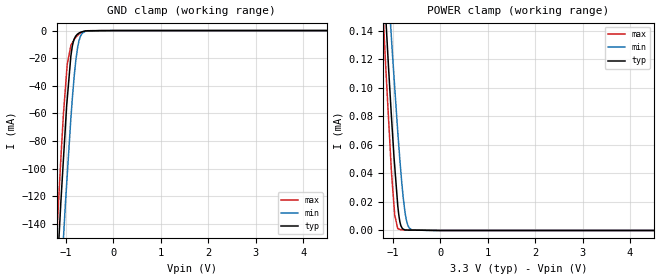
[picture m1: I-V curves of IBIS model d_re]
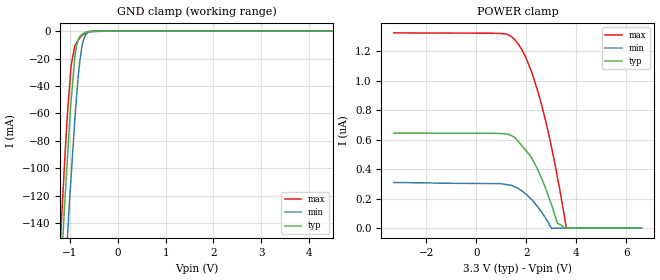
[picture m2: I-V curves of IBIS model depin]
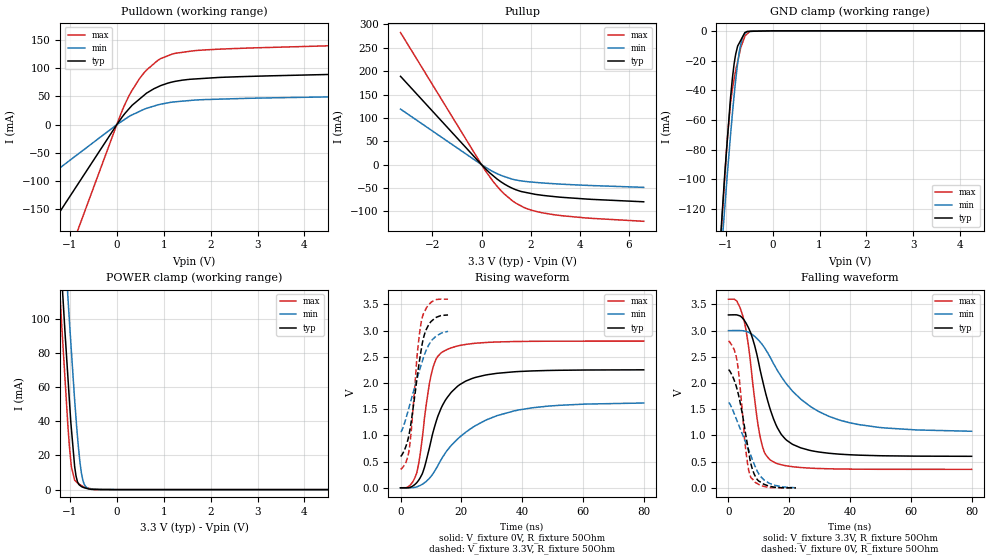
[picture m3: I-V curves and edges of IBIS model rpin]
|Texas Instruments Incorporated
| Low-Power 3.3V-supply Full-Duplex RS-485 Driver / Receiver
| Marketing part#   Digital Voltage Range   Package-type   #pins
| SN65HVD37   3V - 3.6V   D   14
[IBIS Ver]   3.2
[File name]   sn65hvd37.ibs
|SIMDE Ver   V3.0 - 201101 - RHL4 - Build 457
[File Rev]   1.0
[Date]   7/27/2011
[Source]
| Texas Instruments Incorporated.
| Analog-eLab Design Center, HPA
| 12500 TI Blvd
| Dallas, TX -75243
| e-mail: elab_scm_ibis@list.ti.com
[Notes]   Revision History:
| Rev 1.0: 7/27/2011
| - Initial version of the model
| - Model generated from simulations in TISPICE
| - Model matched to SPICE simulation
| - C_comp although listed in numerical order of value are
|   obtained from varying PVT conditions. For PVT conditions for
|   each specific value refer the buffer description under
|   respective [Model]. IBIS model user is responsible for using
|   appropriate C_comp to simulate for Signal Integrity.
|*  EXCEPTION:   *
|*  - For model d_re, there will be a leakage current in the GND   *
|*   clamp I-V Table because of the pullup on pad.   *
|*  - For model depin, there will be a leakage current in the POWER   *
|*   clamp I-V Table because of the pulldown on pad.   *
|*  - For model a_b, there will be a leakage current in both the POWER  *
|*   and GND clamp I-V Tables because of the resistor network connected*
|*   to pad.   *
|*  - For model y_z_*, there will be a leakage current in the POWER   *
|*   clamp I-V Table because of the pulldown on pad.   *
[Disclaimer]
| This model is designed as an aid for customers of Texas Instruments.
| TI and its licensors and suppliers make no warranties, either expressed
| or implied, with respect to this  model, including the warranties of
| merchantability or fitness for a particular purpose. The model is
| provided solely on an "as is" basis. The entire risk as to its quality
| and performance is with the customer.
[Copyright]
 (C) Copyright 2011 Texas Instruments Incorporated.All rights reserved.
|   SN65HVD37
[Component]   SN65HVD37
[Manufacturer]   TI
[Package]   |14 D   -  package
|   typ   min   max
R_pkg   0.05483   0.04472   0.06530
L_pkg   2.20849nH   1.82325nH   2.81275nH
C_pkg   0.42079pF   0.37741pF   0.52665pF
[Pin]  signal_name   model_name   R_pin   L_pin   C_pin
1   NC   NC   0.00380   1.93586nH  0.49616pF
2   R   rpin   0.06530   2.81275nH  0.52665pF
3   _RE   d_re   0.06113   2.26630nH  0.39911pF
4   DE   depin   0.04472   1.82325nH  0.37741pF
5   D   d_re   0.05000   1.97397nH  0.38079pF
6   GND   gnd   0.04998   2.22003nH  0.43776pF
7   GND   gnd   0.04808   2.88519nH  0.56991pF
8   NC   NC   0.00380   1.93586nH  0.49616pF
9   Y   y_z_p   0.06286   2.75675nH  0.52490pF
10   Z   y_z_n   0.05646   2.14750nH  0.39320pF
11   B   a_b   0.04527   1.84090nH  0.37881pF
12   A   a_b   0.05294   2.04647nH  0.38548pF
13   VCC   power   0.05016   2.21543nH  0.43689pF
14   VCC   power   0.04818   2.87772nH  0.56924pF
[Diff_pin]   inv_pin   vdiff   tdelay_typ   tdelay_min   tdelay_max
12   11   80mV   NA   NA   NA
9   10   NA   0   0   0
| Models and submodels in the file (6): d_re (Input), depin (Input), rpin (3-state), a_b (Input), y_z_p (3-state), y_z_n (3-state)
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|   d_re Model
[Model]   d_re
Model_type   Input
Vinl = 0.8
Vinh = 2
|   typ   min   max
|   (nom PVT)   (fast PVT)   (slow PVT)
|C_comp from frequency sweep method (F=10MHz)
|Average
|C_comp   2.050e-12   1.874e-12   2.235e-12
|C_comp from LC tank measurement(L=1nH)
|Average
|Resonant Frequency(Hz)   5.770e+09   5.890e+09   5.550e+09
C_comp   7.616e-13   7.309e-13   8.232e-13
| Where nom  PVT is Nominal Process, 3.3V, 27C
|   Fast PVT is Strong Process,  3.6V, -40C
|   Slow PVT is Weak Process,   3V, 125C
[Voltage Range]   3.3   3   3.6
|Ambient Temperature   25   85   -40
|Junction Temperature
[Temperature Range]   27   125   -40
[Power Clamp Reference]   3.3   3   3.6
[GND Clamp Reference]   0   0   0
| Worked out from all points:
|   GND clamp passes 1 mA (typ) near -0.67 V on its own axis
[GND Clamp]
|   Voltage   I(typ)   I(min)   I(max)
-3.3V     -1.705A    -1.7A      -1.738A
-1.195V   -180.4mA   -237.2mA   -148.9mA
-1.158V   -156.2mA   -213.2mA   -124.7mA
-1.112V   -126.4mA   -185.5mA   -94.94mA
-1.055V   -93.52mA   -150.9mA   -60.84mA
-975.6mV  -50.1mA    -105.4mA   -24.74mA
-897.6mV  -18.42mA   -63.54mA   -10.82mA
-858mV    -9.845mA   -45.32mA   -8.298mA
-792mV    -3.841mA   -21.25mA   -4.834mA
-693mV    -1.195mA   -3.902mA   -1.803mA
-285mV    -92.91uA   -1.638uA   -4.138uA
6.6V      0A         0A         0A
[POWER Clamp]
|   Voltage   I(typ)   I(min)   I(max)
-3.3V     1.551mA    1.444mA    1.676mA
-1.27V    222.2uA    263.9uA    196uA
-1.152V   150.7uA    198.8uA    115.5uA
-1.096V   116.7uA    169.1uA    80.94uA
-1.033V   81.39uA    136.3uA    42.71uA
-961.2mV  44.9uA     100.3uA    10.68uA
-896.4mV  17.2uA     68.68uA    1.244uA
-834.9mV  3.692uA    42.35uA    513.2nA
-744mV    365.5nA    12.7uA     396.5nA
-684mV    295nA      3.558uA    356.6nA
-591mV    254.8nA    379nA      305nA
6.6V      0A         0A         0A
|   depin Model
[Model]   depin
Model_type   Input
Vinl = 0.8
Vinh = 2.0
|   typ   min   max
|   (nom PVT)   (fast PVT)   (slow PVT)
|C_comp from frequency sweep method (F=10MHz)
|Average
|C_comp   2.070e-12   1.894e-12   2.257e-12
|C_comp from LC tank measurement(L=1nH)
|Average
|Resonant Frequency(Hz)   5.770e+09   5.890e+09   5.550e+09
C_comp   7.616e-13   7.309e-13   8.232e-13
| Where nom  PVT is Nominal Process, 3.3V, 27C
|   Fast PVT is Strong Process,  3.6V, -40C
|   Slow PVT is Weak Process,   3V, 125C
[Voltage Range]   3.3   3   3.6
|Ambient Temperature   25   85   -40
|Junction Temperature
[Temperature Range]   27   125   -40
[Power Clamp Reference]   3.3   3   3.6
[GND Clamp Reference]   0   0   0
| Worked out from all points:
|   GND clamp passes 1 mA (typ) near -0.67 V on its own axis
[GND Clamp]
|   Voltage   I(typ)   I(min)   I(max)
-3.3V     -1.705A    -1.7A      -1.738A
-1.195V   -180.4mA   -237.2mA   -148.9mA
-1.158V   -156.2mA   -213.2mA   -124.7mA
-1.112V   -126.4mA   -185.5mA   -94.94mA
-1.055V   -93.52mA   -150.9mA   -60.84mA
-975.6mV  -50.1mA    -105.4mA   -24.74mA
-897.6mV  -18.42mA   -63.54mA   -10.82mA
-858mV    -9.846mA   -45.32mA   -8.298mA
-792mV    -3.842mA   -21.26mA   -4.834mA
-693mV    -1.196mA   -3.903mA   -1.803mA
-285mV    -92.82uA   -1.603uA   -3.947uA
6.6V      0A         0A         0A
[POWER Clamp]
|   Voltage   I(typ)   I(min)   I(max)
-3.3V     645nA      310.1nA    1.325uA
939.6mV   642.6nA    301.8nA    1.322uA
1.422V    626.9nA    289.4nA    1.298uA
1.685V    587.5nA    268.5nA    1.248uA
1.948V    534.5nA    236.2nA    1.169uA
2.168V    490.1nA    201.3nA    1.079uA
2.473V    391.4nA    141.5nA    921.2nA
2.736V    286.6nA    77.39nA    753.7nA
3.003V    161.7nA    0A         553nA
3.241V    34.27nA    0A         349.4nA
3.604V    0A         0A         0A
6.6V      0A         0A         0A
|   rpin Model
[Model]   rpin
Model_type   3-state
Polarity   Non-Inverting
Vmeas = 1.65
Vref = 1.65
Cref = 2pF
Rref = 50
|   typ   min   max
|   (nom PVT)   (fast PVT)   (slow PVT)
|C_comp from frequency sweep method (F=10MHz)
|C_comp   1.603e-11   1.111e-11   2.143e-11
|ON state : BUFFER OUTPUT TURNED HIGH
|C_comp   1.603e-11   1.111e-11   2.143e-11
|OFF state: BUFFER IN HIGH IMPEDANCE
|C_comp   2.602e-12   2.593e-12   2.624e-12
|C_comp from LC tank measurement(L=1nH)
|Resonant Frequency(Hz)   3.430e+09   3.680e+09   3.330e+09
C_comp   2.155e-12   1.872e-12   2.187e-12
|ON state : BUFFER OUTPUT TURNED HIGH
|Resonant Frequency(Hz)   3.230e+09   3.510e+09   3.100e+09
|C_comp   2.430e-12   2.058e-12   2.638e-12
|OFF state: BUFFER IN HIGH IMPEDANCE
|Resonant Frequency(Hz)   3.430e+09   3.680e+09   3.330e+09
|C_comp   2.155e-12   1.872e-12   2.187e-12
| Where nom  PVT is Nominal Process, 3.3V, 27C
|   Fast PVT is Strong Process,  3.6V, -40C
|   Slow PVT is Weak Process,   3V, 125C
[Voltage Range]   3.3   3   3.6
|Ambient Temperature   25   85   -40
|Junction Temperature
[Temperature Range]   27   125   -40
[Pullup Reference]   3.3   3   3.6
[Pulldown Reference]   0   0   0
[Power Clamp Reference]   3.3   3   3.6
[GND Clamp Reference]   0   0   0
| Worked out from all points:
|   slope of the pulldown table from 0 to 0.495 V, typ, clamps not added: 10.7 ohm
|   slope of the pullup table from 0 to 0.495 V, typ, clamps not added: 20.1 ohm
|   GND clamp passes 1 mA (typ) near -0.58 V on its own axis
|   POWER clamp passes 1 mA (typ) near -0.68 V on its own axis
|   falling waveform, V_fixture 3.3V, R_fixture 50Ohm: 20-80 % time 7.75ns typ, 17ns min, 4.39ns max; typ from 3.3 V to 0.602 V
|   rising waveform, V_fixture 0V, R_fixture 50Ohm: 20-80 % time 8.24ns typ, 16.9ns min, 4.17ns max; typ from 0 V to 2.25 V
|   rising waveform, V_fixture 3.3V, R_fixture 50Ohm: 20-80 % time 3.98ns typ, 5.87ns min, 2.87ns max; typ from 0.601 V to 3.3 V
|   falling waveform, V_fixture 0V, R_fixture 50Ohm: 20-80 % time 4.23ns typ, 6.74ns min, 2.79ns max; typ from 2.25 V to 0 V
[Pulldown]
|   Voltage   I(typ)   I(min)   I(max)
-3.3V     -419.7mA   -208.4mA   -743.1mA
-3mV      -381.6uA   -189.4uA   -675.5uA
252mV     27.32mA    14.02mA    49.68mA
478.8mV   44.99mA    23.34mA    80.96mA
633.6mV   55.83mA    28.96mA    96.76mA
939.6mV   69.38mA    36.44mA    117.2mA
1.246V    76.81mA    40.58mA    126.5mA
1.706V    81.24mA    43.83mA    131.5mA
4.504V    88.97mA    49.22mA    139.8mA
5.771V    94.29mA    52.65mA    148.7mA
6.214V    101.2mA    53.85mA    158.4mA
6.6V      107.4mA    54.89mA    172.7mA
[GND Clamp]
|   Voltage   I(typ)   I(min)   I(max)
-3.3V     -1.381A    -1.296A    -1.468A
-1.185V   -176.3mA   -190.9mA   -184.7mA
-1.084V   -127.4mA   -146.2mA   -129.9mA
-1.05V    -111.2mA   -131.8mA   -113.4mA
-972mV    -76.61mA   -99.53mA   -75.44mA
-896.4mV  -45.11mA   -70.2mA    -48.56mA
-818.4mV  -21.9mA    -43.18mA   -32.24mA
-745.8mV  -10.35mA   -22.23mA   -20.92mA
-675mV    -6.16mA    -8.405mA   -10.99mA
-597mV    -1.543mA   -1.883mA   -4.219mA
-537.9mV  -393.4uA   -555uA     -1.926mA
6.6V      0A         0A         0A
[Pullup]
|   Voltage   I(typ)   I(min)   I(max)
-3.3V     188.9mA    118.8mA    282.5mA
172.8mV   -9.472mA   -5.689mA   -14.19mA
633.6mV   -30.76mA   -19.2mA    -46.34mA
939.6mV   -41.74mA   -25.53mA   -63.26mA
1.246V    -50.27mA   -30.87mA   -76.8mA
1.554V    -56.44mA   -34.18mA   -86.73mA
1.84V     -59.76mA   -36.14mA   -93.94mA
2.43V     -65.16mA   -38.87mA   -102.4mA
2.934V    -68.1mA    -40.67mA   -106.9mA
4.314V    -73.62mA   -44.27mA   -114.1mA
6.6V      -79.34mA   -48.49mA   -121mA
[POWER Clamp]
|   Voltage   I(typ)   I(min)   I(max)
-3.3V     1.229A     1.25A      1.228A
-1.29V    180.8mA    229.8mA    154.3mA
-1.174V   124.9mA    173.3mA    96.52mA
-1.155V   116mA      164.4mA    88.18mA
-1.044V   66.95mA    113.8mA    38.42mA
-968.4mV  36.07mA    81.65mA    13.56mA
-897.6mV  13.53mA    52.47mA    5.608mA
-816mV    3.519mA    24.46mA    3.432mA
-726mV    1.429mA    5.877mA    1.926mA
-603mV    426uA      622.4uA    849.2uA
-345mV    82.9uA     5.414uA    6.094uA
6.6V      0A         0A         0A
[Ramp]
R_load = 50
|   typ   min   max
dV/dt_r   1.35083/8.21473e-09   0.970748/1.69203e-08   1.67974/4.16898e-09
dV/dt_f   1.61873/7.74056e-09   1.15189/1.69696e-08   1.94818/4.3737e-09
[Falling Waveform]
V_fixture = 3.3V
V_fixture_min = 3V
V_fixture_max = 3.6V
R_fixture = 50Ohm
|   Time   V(typ)   V(min)   V(max)
0s        3.3V       3V         3.6V
2.775ns   3.3V       3.002V     3.561V
5.075ns   3.208V     2.996V     3.205V
6.5ns     3.066V     2.973V     2.745V
7.975ns   2.844V     2.921V     2.005V
10.27ns   2.292V     2.794V     1.02V
13.88ns   1.475V     2.476V     528.1mV
19.13ns   909.3mV    1.98V      420.4mV
33ns      660.5mV    1.366V     364mV
79.97ns   602.1mV    1.08V      353mV
[Rising Waveform]
V_fixture = 0V
V_fixture_min = 0V
V_fixture_max = 0V
R_fixture = 50Ohm
|   Time   V(typ)   V(min)   V(max)
0s        613pV      31.52nV    241.3pV
3ns       6.483mV    -1.229mV   41.5mV
5.325ns   96.81mV    17.66mV    281.5mV
7.5ns     322.2mV    79.52mV    1.123V
9.975ns   882.6mV    213mV      2.129V
11.68ns   1.258V     361.2mV    2.454V
13.82ns   1.576V     582mV      2.594V
21.63ns   2.041V     1.068V     2.738V
37.45ns   2.214V     1.469V     2.791V
79.97ns   2.251V     1.618V     2.8V
[Rising Waveform]
V_fixture = 3.3V
V_fixture_min = 3V
V_fixture_max = 3.6V
R_fixture = 50Ohm
|   Time   V(typ)   V(min)   V(max)
0s        601.3mV    1.07V      353mV
1.85ns    803.8mV    1.337V     494.8mV
2.85ns    1.029V     1.544V     730.8mV
3.65ns    1.316V     1.713V     1.167V
5.525ns   2.143V     2.098V     2.563V
6.35ns    2.468V     2.263V     2.988V
7.15ns    2.755V     2.412V     3.252V
8.3ns     2.999V     2.605V     3.41V
10.05ns   3.175V     2.797V     3.54V
15.62ns   3.299V     2.986V     3.6V
[Falling Waveform]
V_fixture = 0V
V_fixture_min = 0V
V_fixture_max = 0V
R_fixture = 50Ohm
|   Time   V(typ)   V(min)   V(max)
0s        2.252V     1.625V     2.8V
1.85ns    2.061V     1.424V     2.643V
2.875ns   1.875V     1.273V     2.41V
3.725ns   1.666V     1.148V     1.994V
5.7ns     1.012V     863.6mV    725.4mV
6.625ns   697.8mV    728.4mV    347.4mV
7.4ns     456.5mV    610.8mV    195.9mV
9.425ns   162.8mV    326.5mV    84.28mV
11.92ns   63.52mV    141.6mV    23.58mV
22.17ns   235.1uV    1.945mV    98.92uV
